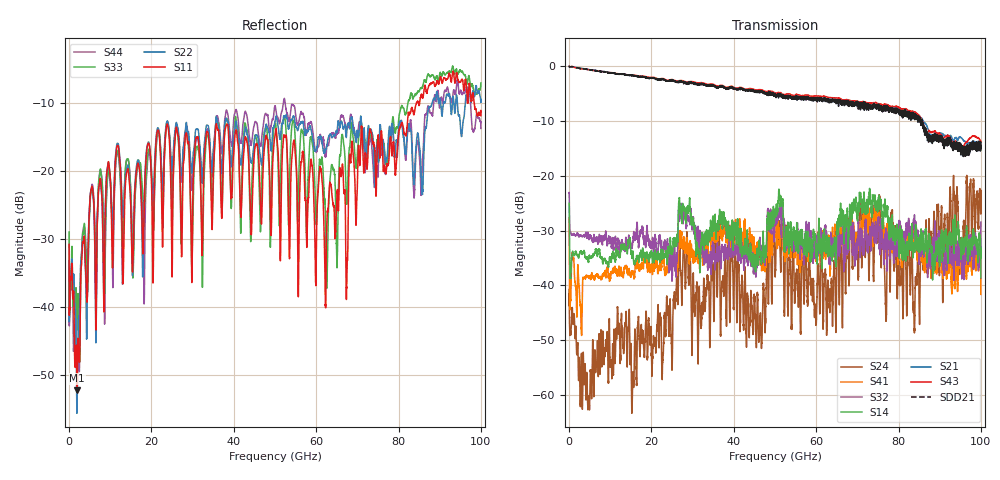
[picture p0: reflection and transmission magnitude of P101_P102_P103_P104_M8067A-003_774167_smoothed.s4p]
!Keysight Technologies PLTS 2021(64 bit), Build 20210202.1
!S11 smoothed in format LOGMAG, average points = 21
!S12 smoothed in format LOGMAG, average points = 21
!S13 smoothed in format LOGMAG, average points = 21
!S14 smoothed in format LOGMAG, average points = 21
!S21 smoothed in format LOGMAG, average points = 21
!S22 smoothed in format LOGMAG, average points = 21
!S23 smoothed in format LOGMAG, average points = 21
!S24 smoothed in format LOGMAG, average points = 21
!S31 smoothed in format LOGMAG, average points = 21
!S32 smoothed in format LOGMAG, average points = 21
!S33 smoothed in format LOGMAG, average points = 21
!S34 smoothed in format LOGMAG, average points = 21
!S41 smoothed in format LOGMAG, average points = 21
!S42 smoothed in format LOGMAG, average points = 21
!S43 smoothed in format LOGMAG, average points = 21
!S44 smoothed in format LOGMAG, average points = 21
!$DUT_CFG_DESC: Default 4-Port Configuration
!$NUMBER_PORTS: 4
!$DIFF_PORT_MAP: 1|2P|2|2P|0|UC|0|UC|
!$PORT_MAP: 1|1|<<<<<<|2|2|>>>>>>|3|3|<<<<<<|4|4|>>>>>>|
!Date: Monday, December 04, 2023, 05:53:19
!S4P File: Measurements: <S11,S12,S13,S14>,
!<S21,S22,S23,S24>,
!<S31,S32,S33,S34>,
!<S41,S42,S43,S44>:
# MHz S  RI  R 50
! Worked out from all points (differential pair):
!   10000 points, 10 MHz to 100 GHz, reference 50 ohm
!   strongest paths, dB at 10 MHz, 25.01 GHz, 50.01 GHz, 75.01 GHz, 100 GHz:
!     S43: 0.0, -2.4, -4.8, -6.8, -13.8
!     S21: 0.0, -2.6, -5.0, -7.3, -14.0
!     S14: -25.0, -34.2, -26.6, -25.7, -38.6
!     S32: -23.2, -38.7, -27.4, -27.9, -28.4
!     S41: -27.7, -36.7, -29.0, -27.9, -41.6
!     S24: -40.8, -54.9, -37.4, -30.0, -26.9
!   taken as a pair (ports 3,1 in; 4,2 out), SDD21 dB: 0.0, -2.6, -5.4, -7.1, -14.9
!   lowest |S11| = -52.3 dB at 1.94 GHz (marker M1), VSWR 1.00, Z = 50.2 + j0.048 ohm
!   |S11| at or under -10 dB: start of sweep to 84.39 GHz; 84.8004 GHz to 85.12949 GHz (329.1 MHz wide, 0.387 % of centre); 98.38 GHz to end of sweep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
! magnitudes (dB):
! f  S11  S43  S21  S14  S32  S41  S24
! 10 MHz  -30.8  0.0  0.0  -25.0  -23.2  -27.7  -40.8
! 1.94 GHz  -52.3  -0.3  -0.2  -34.4  -30.5  -44.2  -52.4
! 5.37 GHz  -22.8  -0.7  -0.6  -35.0  -31.3  -38.5  -58.3
! 11.75 GHz  -16.3  -1.3  -1.4  -34.2  -31.7  -38.0  -44.0
! 52.19 GHz  -14.8  -5.1  -5.3  -32.4  -29.5  -33.5  -42.3
! 62.58 GHz  -27.9  -5.6  -5.9  -32.2  -31.3  -32.6  -48.1
! 100 GHz  -11.9  -13.8  -14.0  -38.6  -28.4  -41.6  -26.9
